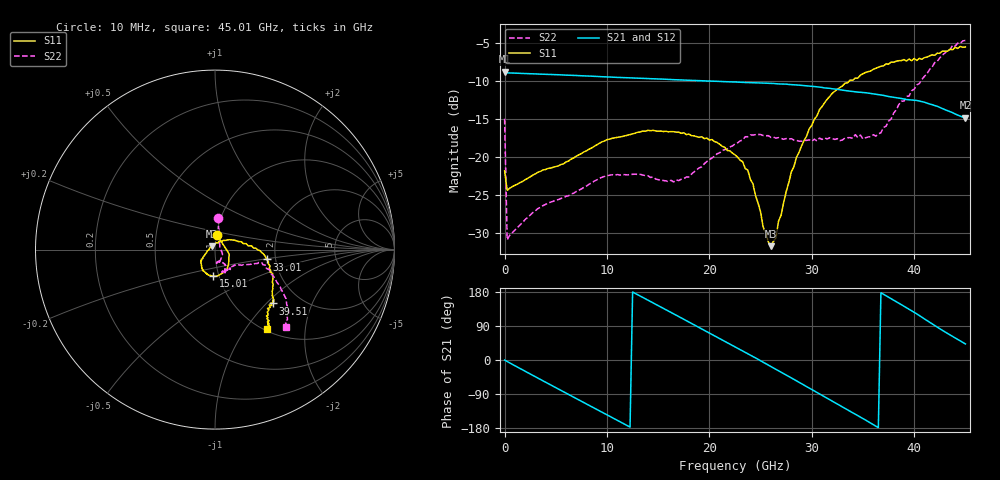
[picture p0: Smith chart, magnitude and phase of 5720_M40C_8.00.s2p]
! Device:  ADRF5720
! Description: 0.5dB LSB GaAs MMIC 6-bit Digital Attenuator
! Frequency:  0.000009 -  40 GHz
! Ports:
!	RF1	= Port 1
!	RF2	= Port 2
! Vdd:  3.3 Volt
! Vss:  -3.3 Volt
! Control:  0/3.3 Volt
! State:  8.00 dB attenuation
! Data:  The device was measured using G-S-G Probes on a matrix board.
!  Data was collected using an calibrated 4 port network analyzer.
!  The reference plane for this measurement is at the launchers.
! Note:  Analog Devices supplies this data as a sample of measured data
!  for this product.  Your particular data for this product may vary.
!  Data was taken at -40 degrees C.
!  Analog Devices reserves the right to change this data at anytime.
# GHZ S DB R 45.0
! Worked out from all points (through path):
!   181 points, 10 MHz to 45.01 GHz, reference 45 ohm
!   highest |S21| = -8.77 dB at 10 MHz (marker M1); lowest = -14.8 dB at 45.01 GHz (marker M2)
!   group delay of S21, straight-line fit = 41.4 ps
!   lowest |S11| = -31.8 dB at 26.01 GHz (marker M3), VSWR 1.05, Z = 43.4 + j1.57 ohm
!   |S11| at or under -10 dB: start of sweep to 33.68 GHz
!   |S22| runs from -30.9 to -4.7 dB; largest |S21 - S12| = 0.0014
!   S11 on the Smith chart (normalised r, x): 10 MHz: 1.01, +0.16; 15.01 GHz: 0.94, -0.28; 33.01 GHz: 1.79, -0.22; 39.51 GHz: 1.47, -1.10; 45.01 GHz: 1.03, -1.27
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0.01  -21.85 82.2  -8.77 -0.2  -8.79 -0.2  -14.99 84.7
0.26  -24.42 6.4  -8.93 -4.0  -8.95 -4.0  -30.95 13.4
4.26  -21.53 -19.6  -9.14 -62.2  -9.16 -62.2  -26.09 -33.5
7.76  -19.35 -45.1  -9.33 -112.5  -9.34 -112.6  -24.01 -59.7
11.51  -17.32 -70.3  -9.55 -166.2  -9.57 -166.3  -22.35 -77.6
15.01  -16.62 -94.1  -9.74 143.5  -9.76 143.4  -23.01 -80.8
15.26  -16.60 -95.8  -9.75 139.9  -9.77 139.8  -23.10 -80.4
17.01  -16.75 -106.3  -9.85 114.7  -9.87 114.6  -23.13 -70.8
19.01  -17.43 -117.5  -9.96 85.8  -9.98 85.7  -21.46 -59.6
22.76  -20.03 -142.1  -10.15 31.2  -10.18 31.1  -18.16 -63.1
24.26  -23.54 -151.6  -10.23 9.2  -10.25 9.1  -17.14 -66.9
25.26  -29.26 -177.4  -10.26 -5.8  -10.29 -5.9  -17.19 -69.1
26.01  -31.78 135.2  -10.32 -17.0  -10.34 -17.1  -17.44 -70.6
26.51  -30.72 92.8  -10.36 -24.6  -10.38 -24.8  -17.54 -72.2
28.01  -22.00 40.0  -10.48 -47.2  -10.51 -47.4  -17.61 -72.1
30.26  -15.03 10.8  -10.73 -81.8  -10.76 -82.0  -17.67 -67.4
33.01  -10.65 -10.8  -11.21 -124.1  -11.24 -124.2  -17.77 -56.2
36.26  -8.33 -33.1  -11.75 -174.5  -11.77 -174.7  -17.26 -38.7
37.76  -7.51 -39.7  -12.10 161.7  -12.13 161.5  -15.01 -28.2
39.51  -7.11 -42.8  -12.48 134.3  -12.50 134.1  -11.99 -16.7
42.01  -6.61 -52.2  -13.24 91.1  -13.26 90.9  -7.58 -29.6
45.01  -5.52 -56.5  -14.84 42.5  -14.87 42.3  -4.66 -47.5
